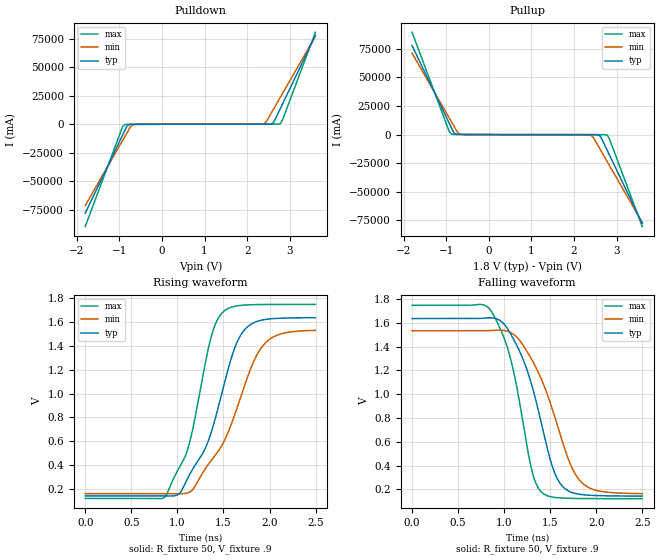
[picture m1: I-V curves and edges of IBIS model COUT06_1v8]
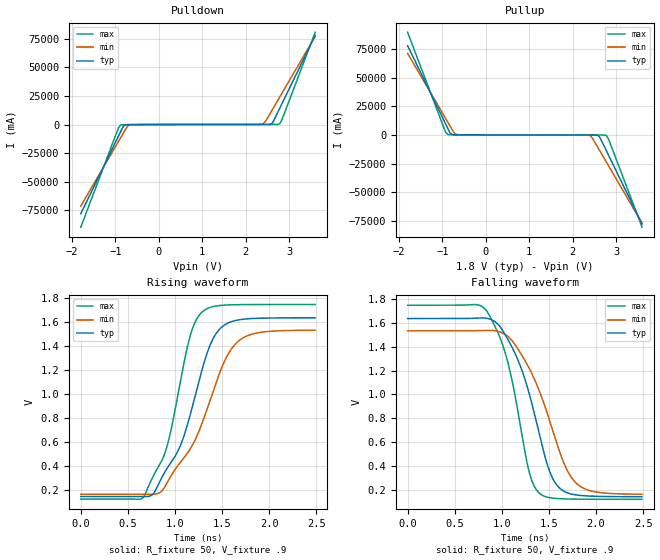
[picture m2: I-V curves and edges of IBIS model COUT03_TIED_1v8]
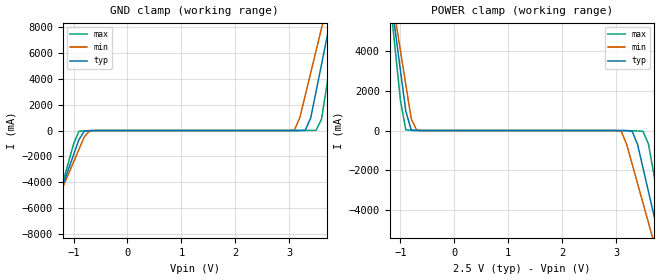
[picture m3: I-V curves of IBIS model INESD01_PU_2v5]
|   This file is an IBIS representation of the   |
|   Integrated Devices Technology, Inc.   |
|   ICS84021   |
|   260MHZ, CRYSTAL-TO-LVCMOS / LVTTL FREQUENCY SYNTHESIZER   |
[IBIS Ver]   4.1
[File name]   84021.ibs
[File Rev]   1.0
[Date]   13 Apr 2009 | Last modified
|   Jun 3 2004 | Generated
[Source]   Originated at Integrated Devices Technology, Inc.
[Disclaimer]
IDT hereby grants the user of this IBIS model a non-exclusive,
nontransferable license to use this IBIS model under the following terms.
Before using this IBIS model, the user should read this license.
If the user does not accept these terms,  the IBIS model should be
returned to IDT within 30 days.
   The user is granted this license only to use the IBIS model and
is not granted rights to sell, load, rent, lease or license the IBIS
model in whole or in part, or in modified form to anyone other than
user. User may modify the IBIS model to suit its specific
applications but rights to derivative works and such modifications
shall belong to IDT.
   This IBIS model is provided on an "AS IS" basis and IDT makes
absolutely no warranty with respect to the information contained
herein. IDT DISCLAIMS AND CUSTOMER WAIVES ALL WARRANTIES, EXPRESS
OR IMPLIED, INCLUDING WARRANTIES OF MERCHANTABILITY OR FITNESS FOR
A PARTICULAR PURPOSE. The entire risk as to quality and performance
is with the Customer. ACCORDINGLY, IN NO EVENT SHALL THE COMPANY BE
LIABLE FOR ANY DAMAGES, WHETHER IN CONTRACT OR TORT,INCLUDING ANY
LOST PROFITS OR OTHER INCIDENTAL, CONSEQUENTIAL, EXEMPLARY, OR
PUNITIVE DAMAGES ARISING OUT OF THE USE OR APPLICATION OF THE IBIS
model provided in this package. Further, IDT reserves the right to
make changes without notice to any product herein to improve
reliability, function, or design. IDT does not convey any license
under patent rights or any other intellectual property rights,
including those of third parties.
   IDT is not obligated to provide maintenance or support
for the licensed IBIS model.
[Copyright]   Copyright 2004 by Integrated Devices Technology, Inc.
[Component]   ICS84021
[Manufacturer] Integrated Devices Technology, Inc.
[Package]
|LQFP32
|lead + wire   typ   min   max
R_pkg   220.4m   212.5m   238m
L_pkg   1.841nH   1.708nH   1.974n
C_pkg   0.316pF   0.2907pF   0.33pF
[Pin]   signal_name   model_name   R_pin   L_pin   C_pin
 1   M5   INESD01_PU   238m   1.974n   0.330p
 2   M6   INESD01_PD   225m   1.841n   0.311p
 3   M7   INESD01_PD   218m   1.7745n   0.301p
 4   M8   INESD01_PD   213m   1.708n   0.291p
 5   N0   INESD01_PD   213m   1.708n   0.291p
 6   N1   INESD01_PD   218m   1.7745n   0.301p
 7   nc   NC   225m   1.841n   0.311p
 8   GND   GND   238m   1.974n   0.330p
 9   TEST   COUT06   238m   1.974n   0.330p
 10   VDD   POWER   225m   1.841n   0.311p
 11   OE1   INESD01_PU   218m   1.7745n   0.301p
 12   OE0   INESD01_PU   213m   1.708n   0.291p
 13   VDDO   POWER   213m   1.708n   0.291p
 14   Q0   COUT03_TIED   218m   1.7745n   0.301p
 15   Q1   COUT03_TIED   225m   1.841n   0.311p
 16   GND   GND   238m   1.974n   0.330p
 17   MR   INESD01_PD   238m   1.974n   0.330p
 18   S_CLOCK   INESD01_PD   225m   1.841n   0.311p
 19   S_DATA   INESD01_PD   218m   1.7745n   0.301p
 20   S_LOAD   INESD01_PD   213m   1.708n   0.291p
 21   VDDA   POWER   213m   1.708n   0.291p
 22   XTAL_SEL   INESD01_PU   218m   1.7745n   0.301p
 23   TEST_CLK   INESD04_PD_PECL  225m   1.841n   0.311p
 24   XTAL_OUT   NC   238m   1.974n   0.330p
 25   XTAL_IN   NC   238m   1.974n   0.330p
 26   nP_LOAD   INESD01_PD   225m   1.841n   0.311p
 27   VCO_SEL   INESD01_PU   218m   1.7745n   0.301p
 28   M0   INESD01_PD   213m   1.708n   0.291p
 29   M1   INESD01_PD   213m   1.708n   0.291p
 30   M2   INESD01_PD   218m   1.7745n   0.301p
 31   M3   INESD01_PD   225m   1.841n   0.311p
 32   M4   INESD01_PD   238m   1.974n   0.330p
[Model Selector] INESD01_PU
INESD01_PU_2v5  Buffer selection for 2v5
INESD01_PU_3v3  Buffer selection for 3v3
[Model Selector] INESD01_PD
INESD01_PD_2v5  Buffer selection for 2v5
INESD01_PD_3v3  Buffer selection for 3v3
[Model Selector] COUT06
COUT06_1v8  Buffer selection for 1v8
COUT06_2v5  Buffer selection for 2v5
COUT06_3v3  Buffer selection for 3v3
[Model Selector] COUT03_TIED
COUT03_TIED_1v8  Buffer selection for 1v8
COUT03_TIED_2v5  Buffer selection for 2v5
COUT03_TIED_3v3  Buffer selection for 3v3
[Model Selector] INESD04_PD_PECL
INESD04_PD_PECL_2v5  Buffer selection for 2v5
INESD04_PD_PECL_3v3  Buffer selection for 3v3
| Models and submodels in the file (12): COUT06_1v8 (Output), COUT03_TIED_1v8 (Output), INESD01_PU_2v5 (Input), INESD01_PD_2v5 (Input), COUT06_2v5 (Output), COUT03_TIED_2v5 (Output), INESD04_PD_PECL_2v5 (Input), INESD01_PU_3v3 (Input), INESD01_PD_3v3 (Input), COUT06_3v3 (Output), COUT03_TIED_3v3 (Output), INESD04_PD_PECL_3v3 (Input)
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[Model] COUT06_1v8
Model_type   Output
Polarity   Non-Inverting
Vmeas = .9
Rref = 50
Cref = 0
Vref = .9
|   typ   min   max
C_comp   2pF   1.5pF   2.5pF
|   typ   min   max
[Voltage range]  1.8V   1.710V   1.890V
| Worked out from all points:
|   slope of the pulldown table from 0 to 0.27 V, typ, clamps not added: 10.3 ohm
|   slope of the pullup table from 0 to 0.27 V, typ, clamps not added: 11.9 ohm
|   rising waveform, R_fixture 50, V_fixture .9: 20-80 % time 373ps typ, 457ps min, 281ps max; typ from 0.143 V to 1.64 V
|   falling waveform, R_fixture 50, V_fixture .9: 20-80 % time 322ps typ, 383ps min, 253ps max; typ from 1.64 V to 0.143 V
[pulldown]
|Voltage   I (typ)   I (min)   I (max)
-1.8V     -77.88A    -71.2A     -89.55A
-927.3mV  -9.821A    -14.52A    -2.535A
-872.7mV  -5.567A    -10.98A    -279.7mA
-818.2mV  -1.447A    -7.441A    -119.4mA
-709.1mV  -98.56mA   -919.5mA   -92.65mA
-654.5mV  -74.81mA   -208.2mA   -85.34mA
2.4V      58.79mA    507.6mA    70.84mA
2.455V    61.02mA    2.637A     70.98mA
2.618V    1.414A     13.25A     71.57mA
2.782V    14.02A     23.86A     493.4mA
2.836V    18.27A     27.4A      4.385A
3.6V      77.78A     76.94A     80.46A
[pullup]
|Voltage   I (typ)   I (min)   I (max)
-1.8V     77.89A     71.2A      89.57A
-927.3mV  9.823A     14.53A     2.543A
-872.7mV  5.569A     10.98A     287mA
-818.2mV  1.45A      7.444A     126.9mA
-709.1mV  101.7mA    922.5mA    99.62mA
-654.5mV  77.73mA    211.3mA    91.37mA
2.4V      -60.59mA   -515mA     -72.08mA
2.455V    -64.65mA   -2.647A    -72.76mA
2.618V    -1.428A    -13.27A    -79.03mA
2.782V    -14.05A    -23.89A    -515mA
2.836V    -18.3A     -27.43A    -4.411A
3.6V      -77.85A    -77.01A    -80.54A
[Ramp]
|   typ   min   max
dV/dt_r   1.195/0.572n   1.095/0.674n   1.302/0.457n
dV/dt_f   1.199/0.493n   1.099/0.579n   1.306/0.395n
[Rising Waveform]
R_fixture = 50
V_fixture = .9
V_fixture_max = .945
V_fixture_min = .855
C_fixture = 0.0p
| Time   typ   min   max
0s        142.8mV    161.8mV    121.5mV
853.4ps   142.9mV    162.1mV    127.1mV
1.019ns   160.2mV    160.7mV    377.7mV
1.146ns   340.2mV    181.3mV    631.5mV
1.354ns   642.8mV    425.5mV    1.437V
1.484ns   1.007V     567.2mV    1.675V
1.679ns   1.479V     951.7mV    1.738V
1.927ns   1.617V     1.4V       1.746V
2.122ns   1.632V     1.5V       1.747V
2.498ns   1.636V     1.53V      1.747V
[Falling Waveform]
R_fixture = 50
V_fixture = .9
V_fixture_max = .945
V_fixture_min = .855
C_fixture = 0.0p
| Time   typ   min   max
0s        1.636V     1.533V     1.747V
858.4ps   1.642V     1.535V     1.699V
1.034ns   1.553V     1.529V     1.393V
1.161ns   1.37V      1.458V     955mV
1.301ns   1.069V     1.287V     354mV
1.414ns   719.6mV    1.106V     170.1mV
1.584ns   277.5mV    720.2mV    129mV
1.714ns   179.9mV    417.8mV    124.2mV
1.824ns   157.8mV    270.7mV    122.8mV
2.498ns   143.2mV    163.9mV    121.5mV
[Model] COUT03_TIED_1v8
Model_type   Output
Polarity   Non-Inverting
Vmeas = .9
Rref = 50
Cref = 0
Vref = .9
|   typ   min   max
C_comp   2pF   1.5pF   2.5pF
|   typ   min   max
[Voltage range]  1.8V   1.710V   1.890V
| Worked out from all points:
|   slope of the pulldown table from 0 to 0.27 V, typ, clamps not added: 10.3 ohm
|   slope of the pullup table from 0 to 0.27 V, typ, clamps not added: 11.9 ohm
|   rising waveform, R_fixture 50, V_fixture .9: 20-80 % time 370ps typ, 453ps min, 278ps max; typ from 0.143 V to 1.64 V
|   falling waveform, R_fixture 50, V_fixture .9: 20-80 % time 327ps typ, 389ps min, 257ps max; typ from 1.64 V to 0.143 V
[pulldown]
|Voltage   I (typ)   I (min)   I (max)
-1.8V     -77.88A    -71.2A     -89.55A
-927.3mV  -9.821A    -14.52A    -2.535A
-872.7mV  -5.567A    -10.98A    -279.7mA
-818.2mV  -1.447A    -7.441A    -119.4mA
-709.1mV  -98.56mA   -919.5mA   -92.65mA
-654.5mV  -74.81mA   -208.2mA   -85.34mA
2.4V      58.79mA    507.6mA    70.84mA
2.455V    61.02mA    2.637A     70.98mA
2.618V    1.414A     13.25A     71.57mA
2.782V    14.02A     23.86A     493.4mA
2.836V    18.27A     27.4A      4.385A
3.6V      77.78A     76.94A     80.46A
[pullup]
|Voltage   I (typ)   I (min)   I (max)
-1.8V     77.89A     71.2A      89.57A
-927.3mV  9.823A     14.53A     2.543A
-872.7mV  5.569A     10.98A     287mA
-818.2mV  1.45A      7.444A     126.9mA
-709.1mV  101.7mA    922.5mA    99.62mA
-654.5mV  77.73mA    211.3mA    91.37mA
2.4V      -60.59mA   -515mA     -72.08mA
2.455V    -64.65mA   -2.647A    -72.76mA
2.618V    -1.428A    -13.27A    -79.03mA
2.782V    -14.05A    -23.89A    -515mA
2.836V    -18.3A     -27.43A    -4.411A
3.6V      -77.85A    -77.01A    -80.54A
[Ramp]
|   typ   min   max
dV/dt_r   1.195/0.568n   1.097/0.672n   1.302/0.454n
dV/dt_f   1.198/0.499n   1.099/0.587n   1.305/0.4n
[Rising Waveform]
R_fixture = 50
V_fixture = .9
V_fixture_max = .945
V_fixture_min = .855
C_fixture = 0.0p
| Time   typ   min   max
0s        142.8mV    161.8mV    121.5mV
669.8ps   141.6mV    161.9mV    141.9mV
771.9ps   167.8mV    161.3mV    317mV
901.4ps   358.7mV    236.1mV    524.7mV
1.043ns   542.1mV    414.8mV    1.045V
1.17ns    851.2mV    551.4mV    1.508V
1.295ns   1.223V     771mV      1.689V
1.449ns   1.518V     1.122V     1.736V
1.678ns   1.619V     1.444V     1.746V
2.488ns   1.636V     1.533V     1.747V
[Falling Waveform]
R_fixture = 50
V_fixture = .9
V_fixture_max = .945
V_fixture_min = .855
C_fixture = 0.0p
| Time   typ   min   max
0s        1.636V     1.533V     1.747V
844.1ps   1.637V     1.538V     1.693V
1.021ns   1.52V      1.509V     1.386V
1.15ns    1.326V     1.405V     945.8mV
1.287ns   1.015V     1.223V     360mV
1.402ns   652.9mV    1.021V     170.3mV
1.559ns   269.5mV    650.9mV    130mV
1.673ns   183.5mV    397.7mV    124.9mV
1.783ns   159mV      262.2mV    123.1mV
2.488ns   143.1mV    163.6mV    121.5mV
[Model] INESD01_PU_2v5
Model_type   Input
Polarity   Non-Inverting
Vinl = 1.4V
Vinh = 1.85V
|   typ   min   max
C_comp   2pF   1.5pF   2.5pF
|   typ   min   max
[Voltage range]  2.5V   2.375V   2.625V
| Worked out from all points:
|   GND clamp passes 1 mA (typ) near -0.54 V on its own axis
|   POWER clamp passes 1 mA (typ) near -0.66 V on its own axis
[GND_clamp]
|Voltage   I(typ)   I(min)   I(max)
-2.5V     -19.6A     -17.18A    -23.67A
-1.6V     -8.969A    -8.332A    -10.1A
-1.5V     -7.788A    -7.349A    -8.588A
-900mV    -707.1mA   -1.46A     -57.43mA
-700mV    -7.027mA   -24.05mA   -13.28mA
3.1V      199.2uA    53.94mA    11.78uA
3.3V      28.4mA     2.748A     652.4uA
3.5V      3.045A     6.192A     15.72mA
3.6V      5.115A     7.914A     872.4mA
3.7V      7.185A     9.638A     3.52A
3.9V      11.33A     13.09A     8.818A
5V        34.14A     32.07A     37.99A
[POWER_clamp]
|Voltage   I(typ)   I(min)   I(max)
-1.5V     9.257A     9.207A     9.48A
-1.2V     7.185A     7.484A     6.83A
-1.1V     5.115A     5.761A     4.182A
-900mV    976.9mA    2.318A     34.23mA
-700mV    1.582mA    24.31mA    1.044mA
3.1V      -2.107mA   -51.03mA   -534.5uA
3.3V      -35.62mA   -1.705A    -10.86mA
3.5V      -1.886A    -3.666A    -39.41mA
3.6V      -3.066A    -4.647A    -666.9mA
3.8V      -5.426A    -6.612A    -3.684A
3.9V      -6.607A    -7.595A    -5.193A
5V        -19.6A     -18.41A    -21.79A
